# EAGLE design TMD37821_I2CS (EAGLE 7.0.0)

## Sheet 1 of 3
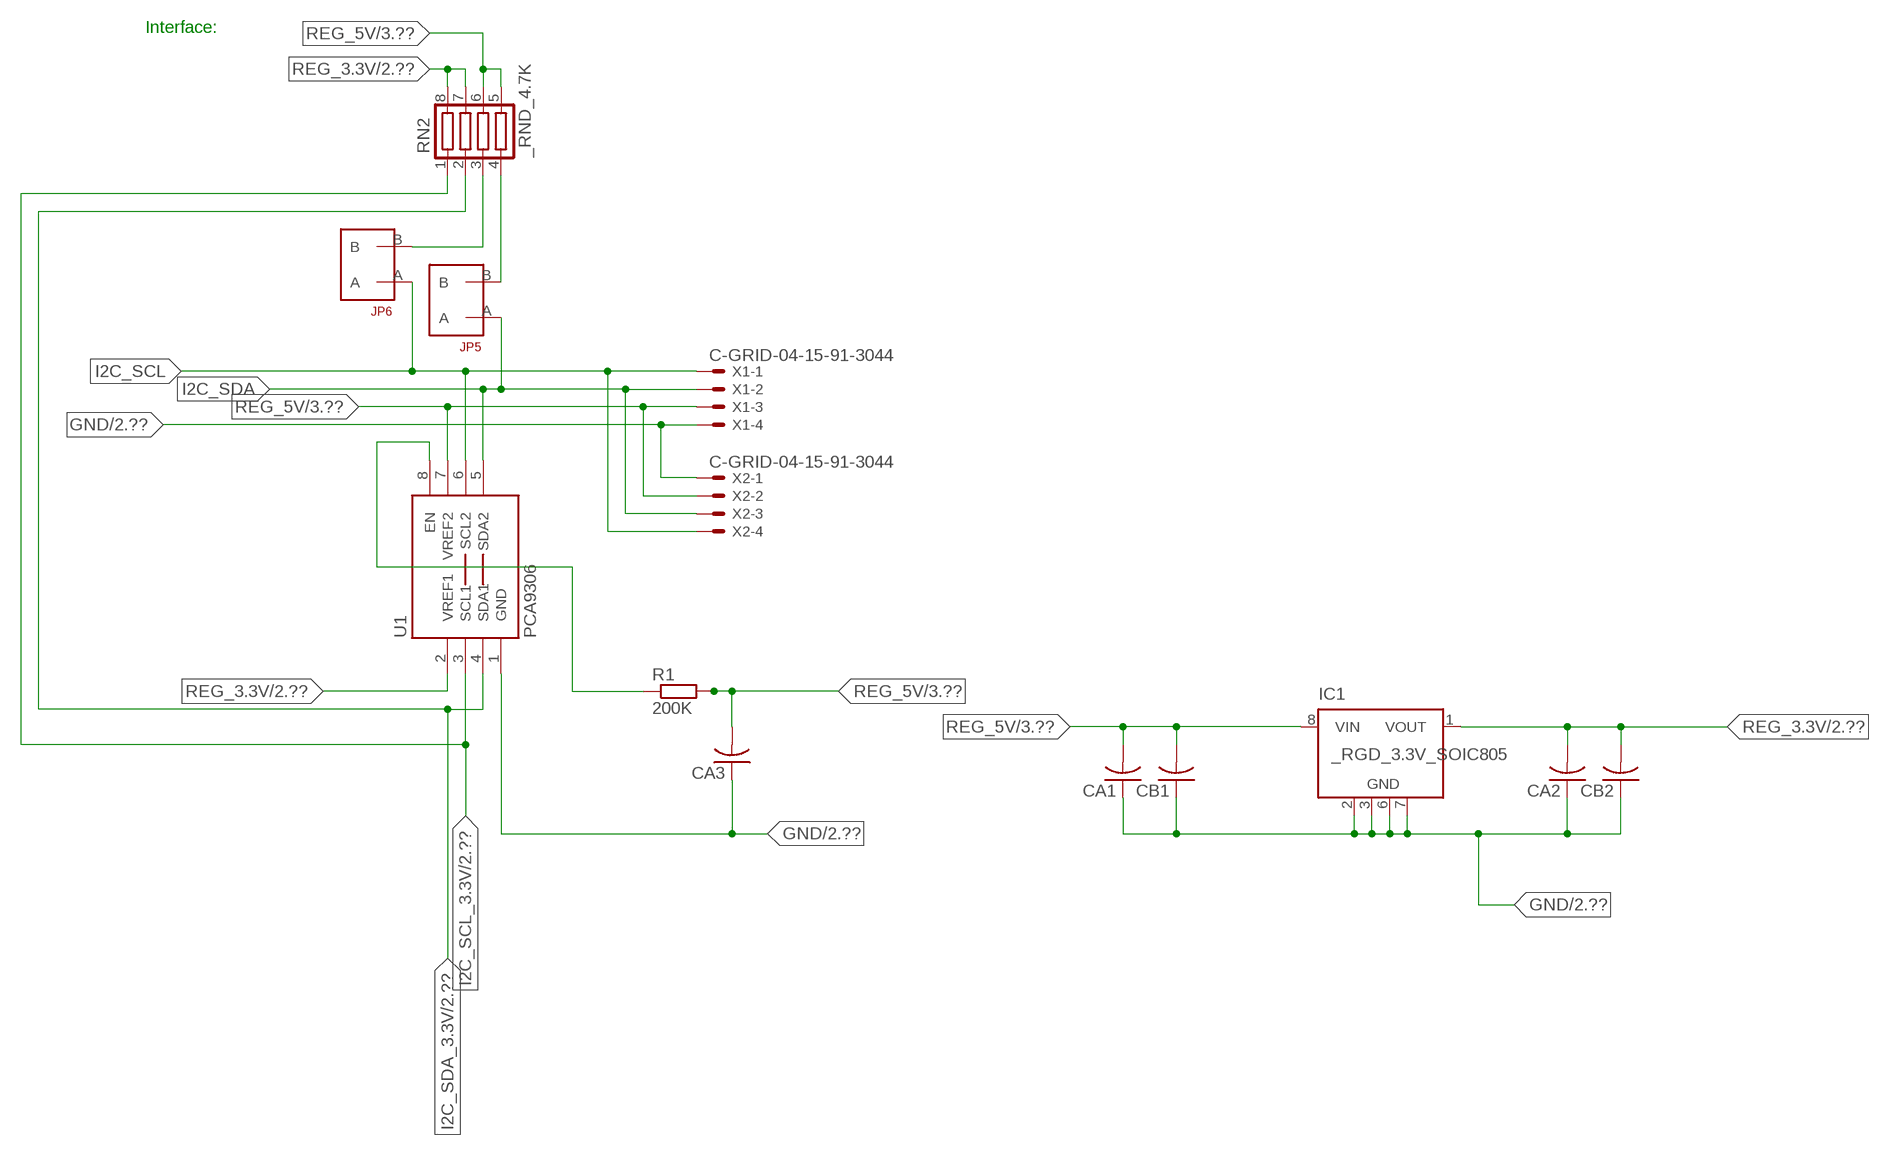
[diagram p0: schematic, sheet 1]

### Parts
CA1  CC1206KRX7R9BB104  [.1UF]
CA2  CC1206KRX7R9BB104  [.1UF]
CA3  CC1206KRX7R9BB104  [.1UF]
CB1  TMK316F106ZL-TC1206K  [TMK316F106ZL-T]
CB2  TMK316F106ZL-TC1206K  [TMK316F106ZL-T]
IC1  _RGD_3.3V_SOIC805  [_RGC_3.3V_SOIC8]
JP5  JUMPER_1X2_2MM  [JUMPER_1X2_2MM]
JP6  JUMPER_1X2_2MM  [JUMPER_1X2_2MM]
R1  200K  RESISTOR_SMT-0603  [R603]
RN2  _RND_4.7K  [RND]
U1  PCA9306  PCA9306_NCD  [PSOP-8]
X1  C-GRID-04-15-91-3044  [15-91-04]
X2  C-GRID-04-15-91-3044  [15-91-04]

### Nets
GND: CA1.1 CA2.1 CA3.1 CB1.1 CB2.1 IC1.2(GND) IC1.3(GND) IC1.6(GND) IC1.7(GND) U1.1(GND) X1.4 X2.1 ; also sheet 2,3
I2C_SCL: JP6.A U1.6(SCL2) X1.1 X2.4
I2C_SCL_3.3V: RN2.1 U1.3(SCL1) ; also sheet 2
I2C_SDA: JP5.A U1.5(SDA2) X1.2 X2.3
I2C_SDA_3.3V: RN2.2 U1.4(SDA1) ; also sheet 2
N$1: JP6.B RN2.3
N$2: JP5.B RN2.4
N$24: R1.1 U1.8(EN)
REG_3.3V: CA2.2 CB2.2 IC1.1(VOUT) RN2.7 RN2.8 U1.2(VREF1) ; also sheet 2
REG_5V: CA1.2 CA3.2 CB1.2 IC1.8(VIN) R1.2 RN2.5 RN2.6 U1.7(VREF2) X1.3 X2.2 ; also sheet 3
Unconnected: IC1.4(NC) IC1.5(NC)

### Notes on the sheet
- Interface:

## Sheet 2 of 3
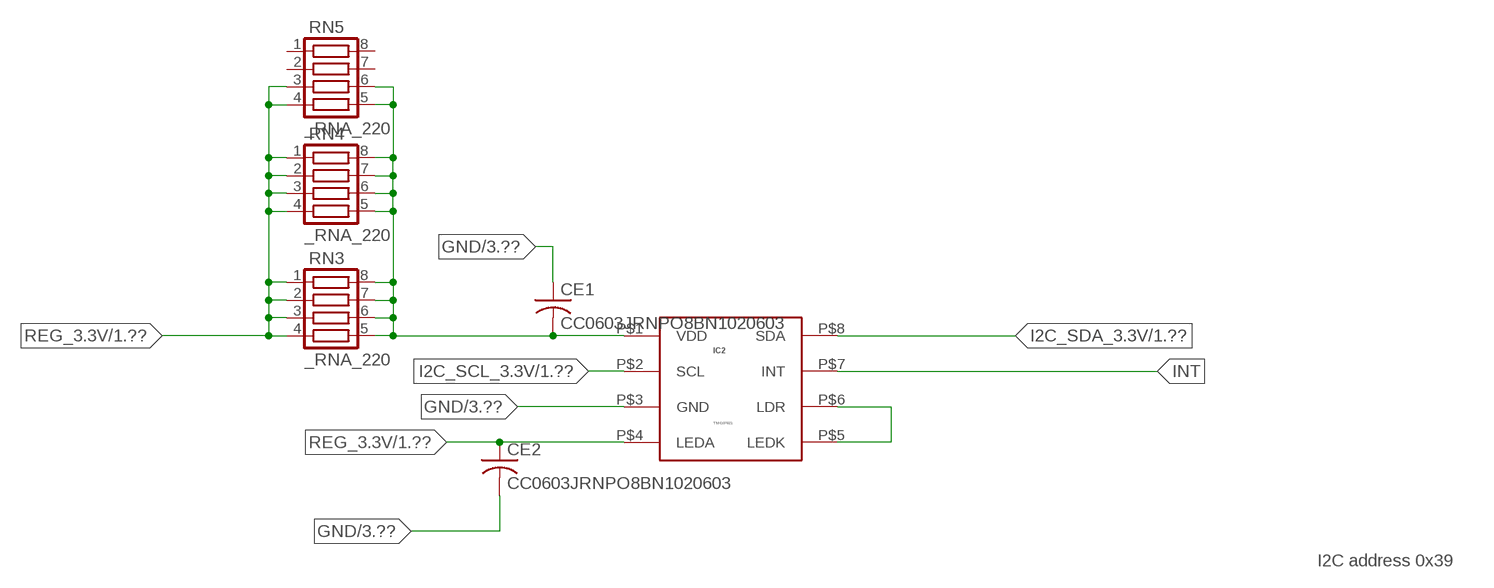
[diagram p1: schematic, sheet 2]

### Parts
CE1  CC0603JRNPO8BN1020603  [CC0603JRNPO8BN102]
CE2  CC0603JRNPO8BN1020603  [CC0603JRNPO8BN102]
IC2  TMD37821  TMD2771  [TMD2771]
RN3  _RNA_220  [RNA]
RN4  _RNA_220  [RNA]
RN5  _RNA_220  [RNA]

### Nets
GND: CE1.1 CE2.2 IC2.P$3(GND) ; also sheet 1,3
I2C_SCL_3.3V: IC2.P$2(SCL) ; also sheet 1
I2C_SDA_3.3V: IC2.P$8(SDA) ; also sheet 1
INT: IC2.P$7(INT)
N$4: IC2.P$5(LEDK) IC2.P$6(LDR)
REG_3.3V: CE2.1 IC2.P$4(LEDA) RN3.1 RN3.2 RN3.3 RN3.4 RN4.1 RN4.2 RN4.3 RN4.4 RN5.3 RN5.4 ; also sheet 1
VDD: CE1.2 IC2.P$1(VDD) RN3.5 RN3.6 RN3.7 RN3.8 RN4.5 RN4.6 RN4.7 RN4.8 RN5.5 RN5.6
Unconnected: RN5.1 RN5.2 RN5.7 RN5.8

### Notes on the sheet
- I2C address 0x39

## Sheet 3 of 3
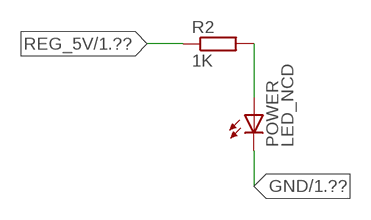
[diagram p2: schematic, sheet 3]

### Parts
POWER  LED_NCD  [CHIPLED_0603]
R2  1K  RESISTOR_SMT-0402  [R402]

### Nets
GND: POWER.C ; also sheet 1,2
N$5: POWER.A R2.2
REG_5V: R2.1 ; also sheet 1

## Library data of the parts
CA1-CA3 = NCD_ULTIMATE_LIBRARY:CC1206KRX7R9BB104: Capacitor CA .1uF 50V SMT C1206K CC1206KRX7R9BB104
CB1 CB2 = NCD_ULTIMATE_LIBRARY:TMK316F106ZL-T: Capacitor CB 10uF SMT 1206 TMK316F106ZL-T
CE1 CE2 = NCD_ULTIMATE_LIBRARY:CC0603JRNPO8BN102: Capacitor CE 1uF SMT CC0603JRNPO8BN102 0603
IC1 = NCD_ULTIMATE_LIBRARY:_RGD_3.3V_SOIC8: Regulator Linear 3.3V Chip Positive VOLTAGE REGULATOR Digikey 497-1199-2-ND/L78L33ACD13TR
IC2 = NCD_ULTIMATE_bhaskar:TMD2771: PROXIMITY DETECTOR DGTL Digikey TMD27711-TTR-ND/TMD27711
JP5 JP6 = NCD_ULTIMATE_CONNECTORS:JUMPER_1X2_2MM
POWER = NCD_ULTIMATE_LIBRARY:LED_NCD: LED Digikey 754-1132-2-ND/APT2012SRCPRV
R1 R2 = NCD_ULTIMATE_LIBRARY:RESISTOR_SMT: NCD Resistor
RN2 = NCD_ULTIMATE_LIBRARY:_RND_4.7K: Resistor Array RND SMT 4.7K x 4 Single Resistor Source: http://www.ctscorp.com/components/Datasheets/CTSChipArrayDs.pdf Digikey 742C083472JPTR-ND/742C083472JP; OC_FARNELL: unknown; OC_NEWARK: unknown
RN3-RN5 = NCD_ULTIMATE_LIBRARY:_RNA_220: Resistor Array RNA SMT 220 x 4 Single Resistor Source: http://www.ctscorp.com/components/Datasheets/CTSChipArrayDs.pdf Digikey 742C083221JPTR-ND/742C083221JP; OC_FARNELL: unknown; OC_NEWARK: unknown
U1 = NCD_ULTIMATE_LIBRARY:PCA9306_NCD: NCD Bidirectional I2C level shifter. NOT compatible with all available part number pinout schemes- DOUBLE CHECK!!!; PROD_ID: IC-10023
X1 X2 = NCD_ULTIMATE_CONNECTORS:C-GRID-04: CONNECTOR 4-Pos I2C wire to board 2.54 mm (0.100") pitch header Digikey WM1342-ND/0015912045; OC_FARNELL: unknown; OC_NEWARK: unknown

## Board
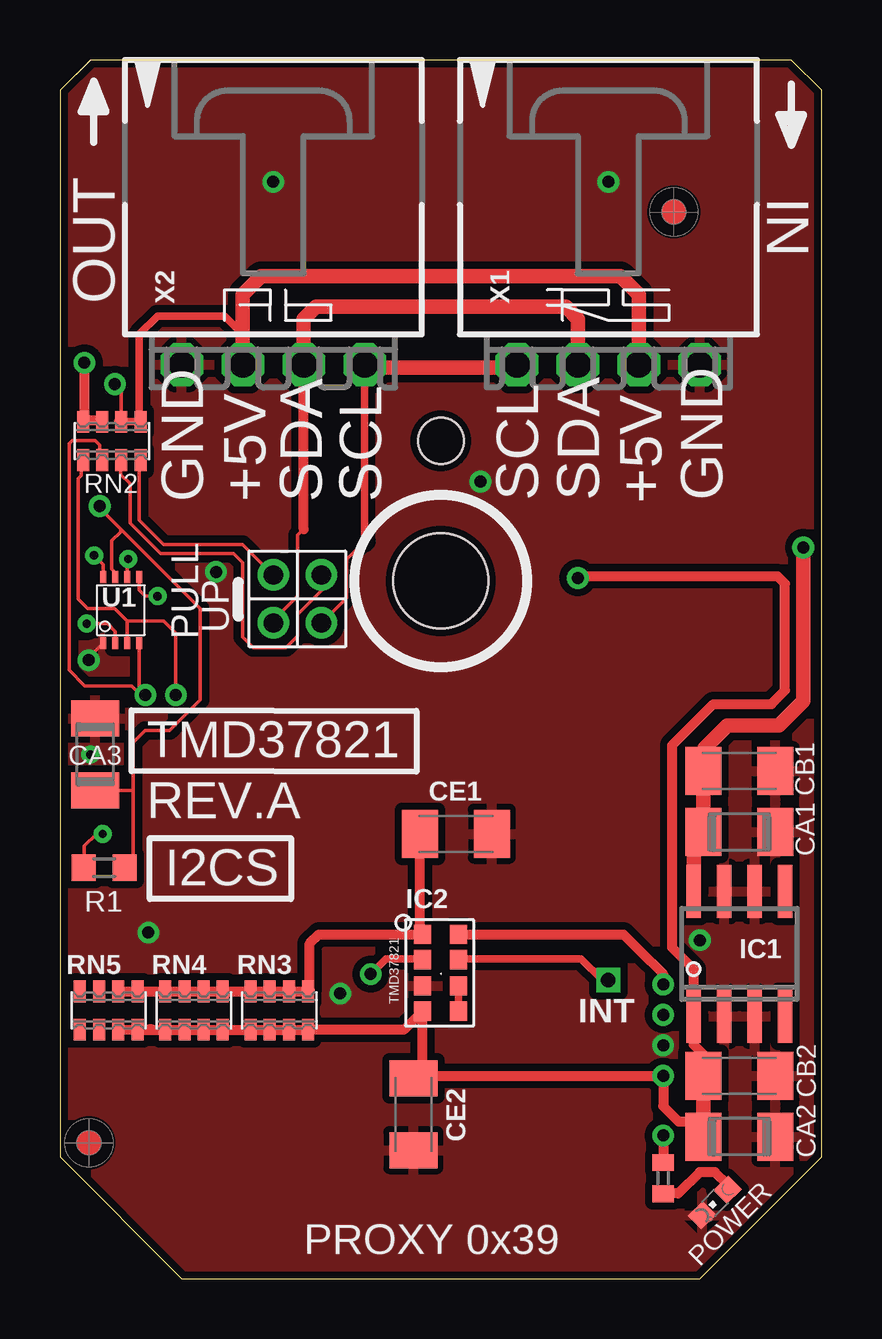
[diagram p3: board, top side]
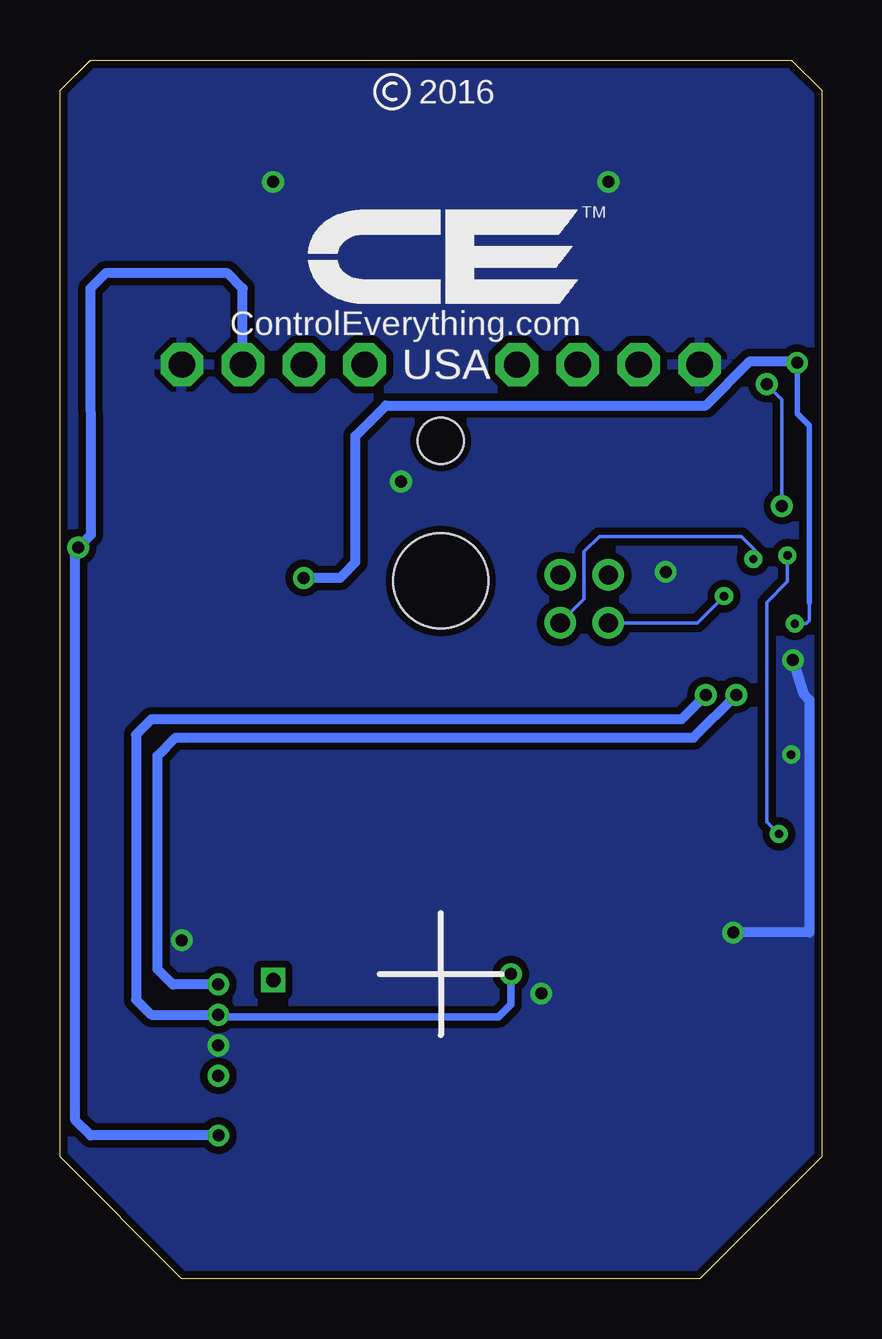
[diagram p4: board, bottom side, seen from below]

Size 31.75 x 50.8 mm. Coordinates in mm from the lower left corner, seen from the top.
Outline: 48 segments
Copper layers (1*16): Top 0.035mm / dielectric 1.5mm / Bottom 0.035mm
Design rules "default": minimum track width 5mil, minimum drill 24mil, track to track 5mil, track to pad 5mil, pad to pad 5mil, via to via 5mil, smd to smd 5mil, copper to edge 10mil, drill to drill 8mil, minimum pad ring 10mil, minimum via ring 8mil, stop-mask expansion 2mil, vias tented up to drill 0mil, thermal gap 10mil
Holes 3.96 mm at 15.88,29.08
Holes 1.91 mm at 15.88,34.93

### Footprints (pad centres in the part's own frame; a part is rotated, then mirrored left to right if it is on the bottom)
.1UF = smd 1.5 x 2: 1 -1.5,0; 2 1.5,0
TMK316F106ZL-T = smd 1.5 x 2: 1 -1.5,0; 2 1.5,0
CC0603JRNPO8BN102 = smd 1.5 x 2: 1 -1.5,0; 2 1.5,0
_RGC_3.3V_SOIC8 = smd 0.6 x 2.2: 1 -1.905,-2.6; 2 -0.635,-2.6; 3 0.635,-2.6; 4 1.905,-2.6; 5 1.905,2.6; 6 0.635,2.6; 7 -0.635,2.6; 8 -1.905,2.6
TMD2771 = smd 0.7 x 0.8: P$1 -2.54,1.905; P$2 -2.54,0.855; P$3 -2.54,-0.245; P$4 -2.54,-1.295; P$5 -1.04,-1.295; P$6 -1.04,-0.245; P$7 -1.04,0.855; P$8 -1.04,1.905
JUMPER_1X2_2MM = drill 0.8: A 0,2; B 0,0
CHIPLED_0603 = smd 0.8 x 0.876: A 0,-0.75; C 0,0.75
R603 = smd 1 x 1.1: 1 -0.85,0; 2 0.85,0
R402 = smd 0.7 x 0.9: 1 -0.65,0; 2 0.65,0
RND = smd 0.5 x 0.9: 1 -1.2,-0.8; 2 -0.4,-0.8; 3 0.4,-0.8; 4 1.2,-0.8; 5 1.2,0.8; 6 0.4,0.8; 7 -0.4,0.8; 8 -1.2,0.8
RNA = smd 0.5 x 0.9: 1 -1.2,-0.8; 2 -0.4,-0.8; 3 0.4,-0.8; 4 1.2,-0.8; 5 1.2,0.8; 6 0.4,0.8; 7 -0.4,0.8; 8 -1.2,0.8
PSOP-8 = smd 0.25 x 0.5: 1 -0.73,-1.37; 2 -0.23,-1.37; 3 0.27,-1.37; 4 0.77,-1.37; 5 0.77,1.38; 6 0.27,1.38; 7 -0.23,1.38; 8 -0.73,1.38
15-91-04 = drill 1.1 pad 1.778 octagon: 1 -3.81,-7.62; 2 -1.27,-7.62; 3 1.27,-7.62; 4 3.81,-7.62

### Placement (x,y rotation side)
CA1  28.32,18.62 180 top
CA2  28.32,5.92 180 top
CA3  1.46,21.86 270 top
CB1  28.32,21.16 180 top
CB2  28.32,8.46 180 top
CE1  16.51,18.54 180 top
CE2  14.73,6.86 270 top
IC1  28.32,13.54 0 top
IC2  17.65,12.45 0 top
JP5  8.89,29.34 180 top
JP6  10.9,29.34 180 top
POWER  27.3,3.18 135 top
R1  1.84,17.13 0 top
R2  25.15,4.19 270 top
RN2  2.16,34.93 0 top
RN3  9.14,11.18 0 top
RN4  5.59,11.18 0 top
RN5  2.03,11.18 0 top
U1  2.54,27.86 0 top
U$5  [VISION_REF10]  1.21,5.66 90 top
U$28  [VISION_REF10]  25.59,44.46 90 top
X1  22.86,45.72 0 top
X2  8.89,45.72 0 top

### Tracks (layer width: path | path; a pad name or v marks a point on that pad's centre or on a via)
GND  (via drill 0.35, 0.5)
  Top 0.152: CA3.1 1.52,23.42 1.52,23.62 | U1.1 1.27,25.96 v1.19,25.78
  Bottom 0.406: v1.19,25.78 0.76,24.38 0.51,24.13 0.51,14.43 v3.69,14.43
  other vias: 8.89,45.72 22.86,45.72 25.15,9.73 17.53,33.22 26.67,14.11 6.5,29.46 11.69,11.89 1.27,21.84
  pour Bottom (isolate 0.305): -0.64,5.08 -0.64,49.53 1.27,51.44 30.48,51.44 32.38,49.53 32.38,5.08 26.67,-0.63 5.08,-0.63
  pour Top (isolate 0.305): 4.45,-1.27 -1.27,4.45 -1.27,50.17 0.64,52.07 31.11,52.07 33.02,50.17 33.02,4.45 27.3,-1.27
I2C_SCL  (via drill 0.35)
  Top 0.152: 12.7,30.73 11.94,29.97 11.94,28.38 JP6.A | v2.85,30 2.81,29.96 U1.6
  Top 0.305: 12.7,30.73 X2.4
  Top 0.406: X2.4 12.7,37.97 | 19.05,37.97 X1.1
  Top 0.61: 12.7,37.97 19.05,37.97
  Bottom 0.152: JP6.A 9.91,28.33 9.91,30.3 9.27,30.94 3.35,30.94 2.79,30.38 v2.85,30
I2C_SCL_3.3V  (via drill 0.5)
  Top 0.152: RN2.1 0.89,34.07 0.89,33.48 0.77,33.35 0.77,28.33 1.16,27.94 2.29,27.94 2.81,27.42 | 2.81,27.42 U1.3 | v4.83,24.33 v4.83,24.34 4.83,26.92 4.33,27.42 2.81,27.42
  Top 0.305: 14.99,13.34 13.59,13.34 v12.95,12.7
  Top 0.406: IC2.P$2 14.99,13.34
  Bottom 0.305: v25.15,11 25.07,10.92 13.46,10.92 12.95,11.43 v12.95,12.7
  Bottom 0.406: v4.83,24.33 5.84,23.32 27.94,23.32 28.58,22.68 28.58,11.63 27.94,11 v25.15,11
I2C_SDA  (via drill 0.35)
  Top 0.152: JP5.A 8.89,27.44 9.91,28.45 9.91,30.99 10.16,31.24 | U1.5 3.3,28.7 3.56,28.45 v4.06,28.45
  Top 0.406: 10.16,31.24 10.16,31.25 X2.3
  Top 0.61: X2.3 10.16,40.01 10.67,40.51 21.09,40.51 21.59,40.01 X1.2
  Bottom 0.152: v4.06,28.45 5.17,27.34 JP5.A
I2C_SDA_3.3V  (via drill 0.5)
  Top 0.152: RN2.2 1.65,34.14 1.65,34.75 1.46,34.94 0.51,34.94 0.38,34.81 0.38,26.37 0.38,26.36 0.38,25.38 1.04,24.71 3,24.71 3.38,24.33 v3.56,24.33 3.31,24.58 U1.4
  Top 0.406: IC2.P$8 23.49,14.35 24.13,13.72 25.15,12.7 v25.15,12.27
  Bottom 0.406: v25.15,12.27 27.05,12.27 27.69,12.9 27.69,21.79 26.93,22.56 5.34,22.56 v3.56,24.33
INT  (via drill 0.6)
  Top 0.305: IC2.P$7 16.8,13.34 21.72,13.34 22.61,12.45 v22.86,12.45
N$1
  Top 0.152: JP6.B 10.92,29.31 10.92,28.7 9.91,27.69 9.91,26.8 9.42,26.31 8.06,26.31 7.62,26.75 7.62,29.84 7.24,30.23 4.19,30.23 2.92,31.5 2.92,33.15 2.54,33.53 2.54,34.1 RN2.3
  Top 0.305: 2.54,34.02 RN2.3
N$2
  Top 0.152: JP5.B 7.62,30.61 4.32,30.61 3.3,31.62 3.3,34.07 RN2.4
  Top 0.305: 3.37,33.88 RN2.4
N$4
  Top 0.305: IC2.P$5 IC2.P$6
N$5
  Top 0.406: POWER.A 27.84,3.92 27.3,4.45 26.67,4.45 25.78,3.56 25.16,3.56 R2.2
N$24  (via drill 0.35)
  Top 0.152: R1.1 1.02,17.16 1.02,18.03 1.52,18.54 v1.78,18.54 | v1.42,30.15 1.81,29.77 U1.8
  Bottom 0.152: v1.78,18.54 2.29,19.05 2.29,28.19 1.42,29.06 v1.42,30.15
REG_3.3V  (via drill 0.35, 0.5)
  Top 0.152: v1.12,27.31 1.98,27.31 2.31,26.98 U1.2
  Top 0.406: CB2.2 26.82,9.35 26.42,9.75 26.42,10.36 | 26.82,6.55 25.78,6.55 25.15,7.19 v25.15,8.46 15.14,8.46 15.11,8.61 | IC1.1 26.42,12.9 25.53,13.79 25.53,22.24 27.24,23.95 29.66,23.95 30.23,24.52 30.23,28.97 29.91,29.29 21.67,29.29 v21.59,29.21 | 26.52,5.62 CA2.2 | v1.02,38.18 1.02,35.78 | 1.02,35.78 RN2.8 | 1.02,35.78 1.71,35.78 RN2.7 | RN5.3 3.74,10.41 3.81,10.41 3.85,10.38 RN5.4 RN4.1 RN4.2 RN4.3 RN4.4 RN3.1 RN3.2 RN3.3 RN3.4 14.34,10.38 IC2.P$4 15.11,8.61 | CE2.1 15.11,8.61
  Top 0.61: CB2.2 26.82,6.55 CA2.2 | 26.42,10.36 IC1.1
  Bottom 0.152: 0.51,28.19 0.51,27.43 0.64,27.31 v1.12,27.31
  Bottom 0.229: 0.51,28.19 0.51,35.56 1.02,36.07 v1.02,38.18
  Bottom 0.406: v1.02,38.18 1.08,38.24 2.99,38.24 4.83,36.4 18.16,36.4 19.43,35.13 19.43,29.87 19.94,29.34 20.07,29.21 v21.59,29.21
REG_5V  (via drill 0.5)
  Top 0.152: RN2.6 2.56,37.01 v2.29,37.29 | R1.2 3.05,17.49 3.05,20.36 | 3.05,20.36 3.05,22.35 3.56,22.86 4.57,22.86 5.84,24.13 5.84,27.94 2.53,31.26 | CA3.2 3.05,20.36 | 2.53,31.26 1.65,32.13 v1.65,32.21 | U1.7 2.29,29.27 2.29,29.46 2.16,29.59 2.16,30.76 2.53,31.13 2.53,31.26
  Top 0.305: 7.62,39.37 7.5,39.37 | 2.42,35.74 RN2.6 RN2.5 3.31,35.8 3.31,39.37 4.07,40.13 6.86,40.13 7.62,39.37 | X2.2 7.62,39.37
  Top 0.406: v25.15,5.97 R2.1
  Top 0.61: X1.3 24.13,41.02 23.37,41.78 8.38,41.78 7.62,41.02 X2.2 | IC1.8 26.42,18.21 CA1.2 CB1.2 26.86,21.2 26.86,22.11 27.82,23.06 29.98,23.06 30.99,24.08 v30.99,30.48
  Bottom 0.152: v1.65,32.21 1.65,36.65 v2.29,37.29
  Bottom 0.406: X1.3 24.13,41.28 24.77,41.91 29.85,41.91 30.48,41.27 30.47,31 v30.99,30.48 31.11,30.36 31.11,6.6 30.48,5.97 v25.15,5.97
VDD
  Top 0.406: RN5.6 RN5.5 RN4.8 RN4.7 RN4.6 RN4.5 RN3.8 RN3.7 RN3.6 RN3.5 10.41,12.05 10.41,13.97 10.79,14.35 IC2.P$1 15.01,14.5 CE1.2

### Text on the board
tNames: IN | OUT | GND | +5V | SDA | SCL | SCL | SDA | +5V | GND | PULL | UP | TMD37821 | REV.A | I2CS | INT | PROXY 0x39
bNames: 2016 | TM | ControlEverything.com | USA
